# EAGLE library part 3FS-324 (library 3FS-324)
Power Transformers POWER TRANSFORMER Source: Datasheet
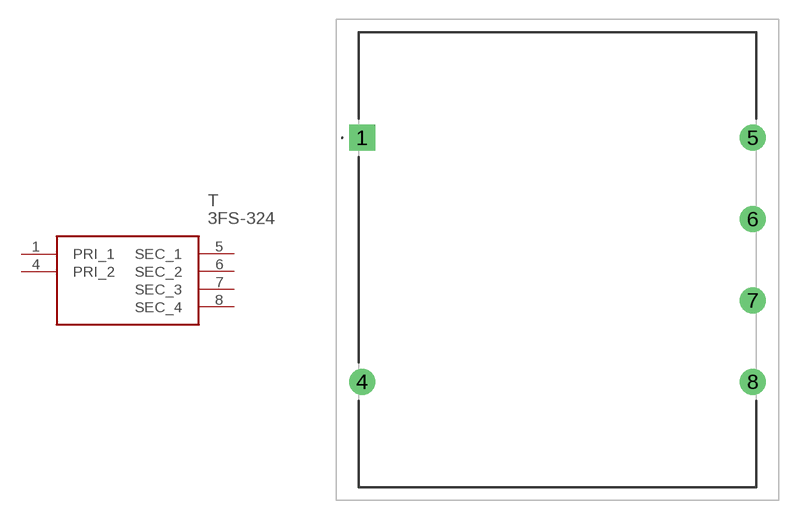
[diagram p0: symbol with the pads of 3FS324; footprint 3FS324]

Designator prefix T

## 3FS-324 (Description: Power Transformers POWER TRANSFORMER; Height: 32.1mm; Manufacturer_Name: Tamura; Manufacturer_Part_Number: 3FS-324; Mouser_Part_Number: 838-3FS-324; Mouser_Price-Stock: https://www.mouser.com/Search/Refine.aspx?Keyword=838-3FS-324)  [3FS324]
1  PRI_1
4  PRI_2
5  SEC_1
6  SEC_2
7  SEC_3
8  SEC_4

## Footprint 3FS324 (pad centres in mm)
3FS-324-1
drill 1.35 pad 2.025 square: 1 0,0
drill 1.35 pad 2.025: 4 0,-19.05; 5 30.48,0; 6 30.48,-6.35; 7 30.48,-12.7; 8 30.48,-19.05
